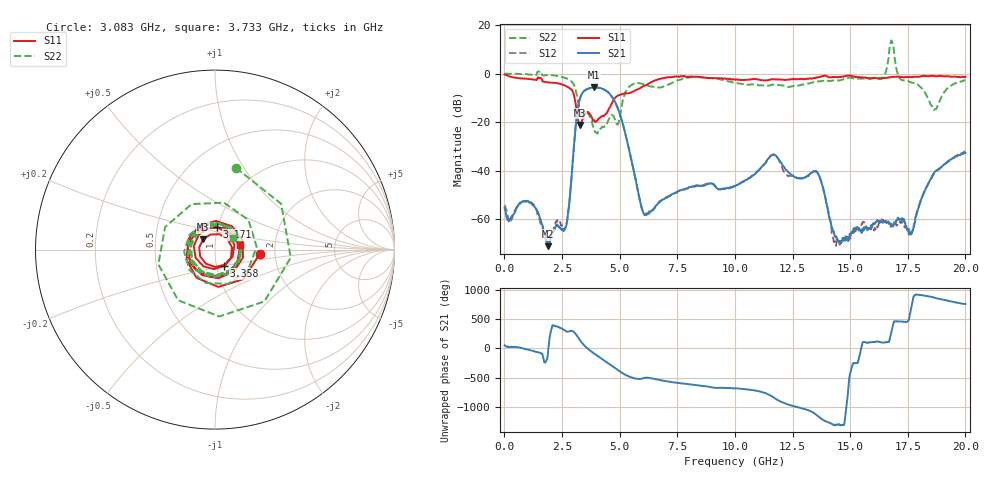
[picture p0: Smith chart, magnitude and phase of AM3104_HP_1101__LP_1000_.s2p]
!Created with skrf (http://scikit-rf.org).
# Hz S RI R 50.0
!freq ReS11 ImS11 ReS21 ImS21 ReS12 ImS12 ReS22 ImS22
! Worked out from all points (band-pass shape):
!   1601 points, 10 MHz to 20 GHz, reference 50 ohm
!   highest |S21| = -5.69 dB at 3.883 GHz (marker M1); lowest = -71.1 dB at 1.884 GHz (marker M2)
!   |S21| within 3 dB of the highest: 3.344 GHz to 4.603 GHz (1.259 GHz wide, 31.7 % of centre)
!   lowest |S11| = -21.2 dB at 3.283 GHz (marker M3), VSWR 1.19, Z = 43.5 + j4.99 ohm
!   |S11| at or under -10 dB: 3.045 GHz to 4.8 GHz (1.755 GHz wide, 44.7 % of centre)
!   |S22| runs from -24.7 to 13.6 dB; largest |S21 - S12| = 0.041
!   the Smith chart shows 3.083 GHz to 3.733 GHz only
!   S11 on the Smith chart (normalised r, x): 3.083 GHz: 1.66, -0.08; 3.171 GHz: 0.99, +0.25; 3.358 GHz: 1.09, -0.20; 3.733 GHz: 1.32, +0.08
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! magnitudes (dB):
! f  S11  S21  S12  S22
! 10 MHz  -0.4  -55.4  -54.2  0.0
! 1.122 GHz  -2.2  -53.2  -53.1  -0.4
! 1.884 GHz  -3.6  -71.1  -68.4  -0.7
! 2.671 GHz  -5.1  -63.0  -62.2  -1.9
! 3.083 GHz  -12.0  -22.7  -22.7  -6.6
! 3.171 GHz  -18.0  -15.4  -15.5  -10.3
! 3.283 GHz  -21.2  -10.1  -10.2  -15.3
! 3.346 GHz  -20.1  -8.6  -8.7  -16.8
! 3.358 GHz  -19.7  -8.4  -8.5  -16.9
! 3.733 GHz  -17.0  -5.8  -5.9  -18.3
! 3.883 GHz  -19.2  -5.7  -5.7  -22.5
! 4.895 GHz  -9.2  -13.7  -13.7  -21.0
! 6.044 GHz  -5.1  -57.7  -57.3  -4.4
! 6.682 GHz  -2.3  -53.3  -53.4  -5.7
! 10.01 GHz  -2.5  -46.4  -46.5  -3.9
! 11.65 GHz  -2.4  -33.4  -33.4  -4.5
! 13.34 GHz  -2.1  -40.8  -40.8  -3.8
! 14.37 GHz  -1.4  -67.4  -70.1  -2.8
! 16.68 GHz  -1.6  -61.5  -62.2  7.2
! 17.65 GHz  -1.4  -66.0  -66.3  -3.7
! 18.66 GHz  -1.0  -40.6  -40.8  -14.7
! 20 GHz  -1.3  -32.7  -32.1  -2.8
